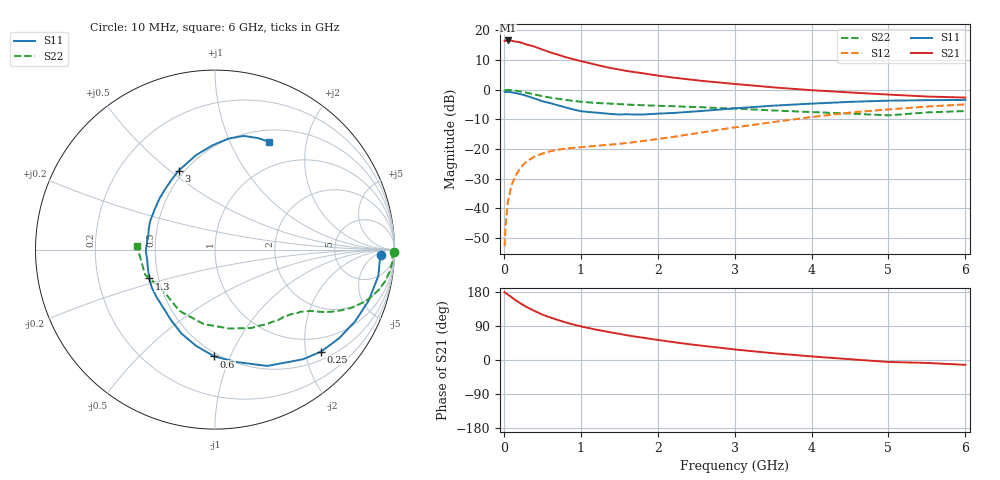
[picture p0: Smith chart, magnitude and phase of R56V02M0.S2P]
! SIEMENS Small Signal Semiconductors
! BFR183
! Si NPN RF Bipolar Junction Transistor in SOT23
! VCE = 6 V  IC = 2 mA
! Common Emitter S-Parameters:  May  1996
# GHz  S  MA  R  50
!  f  S11  S21  S12  S22
! GHz  MAG  ANG  MAG  ANG  MAG  ANG  MAG  ANG
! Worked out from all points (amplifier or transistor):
!   36 points, 10 MHz to 6 GHz, reference 50 ohm
!   highest |S21| = 16.6 dB at 50 MHz (marker M1)
!   |S21| within 3 dB of that: start of sweep to 492.5 MHz
!   unconditionally stable (mu >= 1): 1.411 GHz to 2.836 GHz
!   at 250 MHz: K = 0.22, MSG = 20.5 dB, |S12| = -25.4 dB
!   at 1.4 GHz: K = 1.00, MSG = 12.9 dB, |S12| = -18.5 dB
!   at 6 GHz: K = 0.90, MSG = 1.1 dB, |S12| = -5.0 dB
!   S11 on the Smith chart (normalised r, x): 10 MHz: 22, -9; 250 MHz: 0.67, -2.32; 600 MHz: 0.47, -0.87; 1.3 GHz: 0.44, -0.17; 3 GHz: 0.47, +0.54; 6 GHz: 0.65, +1.42
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0.01  0.9243 -1.8  6.716 178.8  0.0023 88.8  0.996 -0.7
0.02  0.92 -3.9  6.604 176.9  0.0048 92.1  0.9861 -1.4
0.05  0.9219 -9.1  6.759 172.8  0.0124 84.3  0.9924 -3.7
0.1  0.9024 -18.3  6.694 165.9  0.0245 80.2  0.9803 -7.3
0.15  0.8771 -27.1  6.478 158.2  0.0351 74.9  0.9629 -10.7
0.2  0.8498 -35.5  6.355 151.6  0.0449 70.3  0.9394 -13.8
0.25  0.8204 -43.8  6.067 145.3  0.054 66.3  0.9115 -16.6
0.3  0.7831 -51.3  5.762 139.5  0.0622 62.8  0.8866 -18.9
0.4  0.7106 -65.8  5.306 129.4  0.0746 56.6  0.8305 -22.9
0.5  0.6382 -79.1  4.745 119.8  0.0836 52.0  0.7767 -25.9
0.6  0.5952 -90.4  4.279 112.5  0.0914 48.3  0.7368 -28.0
0.8  0.5039 -111.7  3.546 99.4  0.1015 44.1  0.6743 -30.9
0.9  0.4643 -121.6  3.277 93.8  0.1047 43.3  0.6471 -32.0
1.1  0.4202 -140.5  2.826 84.4  0.1102 43.3  0.6113 -34.2
1.3  0.3995 -156.3  2.455 76.3  0.1162 44.0  0.5877 -36.2
1.7  0.3809 173.0  1.977 62.1  0.1308 48.3  0.5529 -40.8
2.2  0.4047 145.9  1.6 47.3  0.1599 52.9  0.5271 -48.2
3  0.4841 114.7  1.25 27.9  0.2311 54.3  0.4814 -65.2
3.5  0.5376 101.2  1.095 17.9  0.2844 51.1  0.4464 -79.9
4.5  0.6233 83.0  0.898 2.1  0.4113 39.7  0.3946 -120.2
5.5  0.6655 69.0  0.767 -7.7  0.5195 25.3  0.4137 -160.3
6  0.6721 63.3  0.736 -12.8  0.5654 16.1  0.4363 177.1
